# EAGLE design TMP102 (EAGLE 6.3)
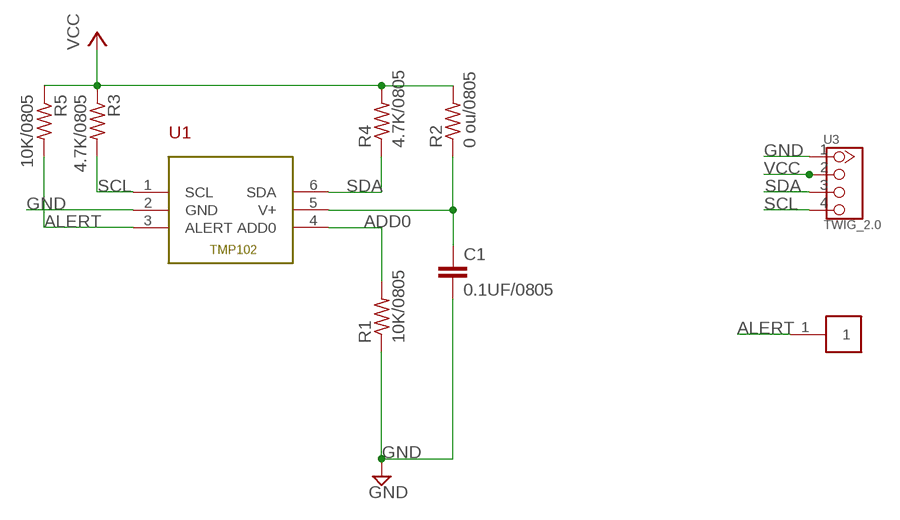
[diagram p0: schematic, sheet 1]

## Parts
C1  0.1UF/0805  C-EUC0805  [C0805]
R1  10K/0805  R-US_R0805  [R0805]
R2  0 ou/0805  R-US_R0805  [R0805]
R3  4.7K/0805  R-US_R0805  [R0805]
R4  4.7K/0805  R-US_R0805  [R0805]
R5  10K/0805  R-US_R0805  [R0805]
U1  TMP102  [TMP102]
U3  TWIG_2.0  [2.0_1X4]
U$1  PIN-1-2.0  [PIN-1-2.0]

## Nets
ADD0: R1.2 U1.4(ADD0)
ALERT: R5.2 U1.3(ALERT) U$1.1
GND: C1.2 R1.1 U1.2(GND) U3.1
N$6: C1.1 R2.1 U1.5(V+)
SCL: R3.2 U1.1(SCL) U3.4
SDA: R4.1 U1.6(SDA) U3.3
VCC: R2.2 R3.1 R4.2 R5.1 U3.2

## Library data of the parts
C1 = resistor:C-EU: CAPACITOR, European symbol
R1-R5 = resistor:R-US_: RESISTOR, American symbol
U1 = TMP102:TMP102
U3 = CONNECTER:TWIG_2.0
U$1 = PIN-1-2.0:PIN-1-2.0

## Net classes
0 default: width 0.003 mm, drill 0.254 mm, clearance 0.152 mm

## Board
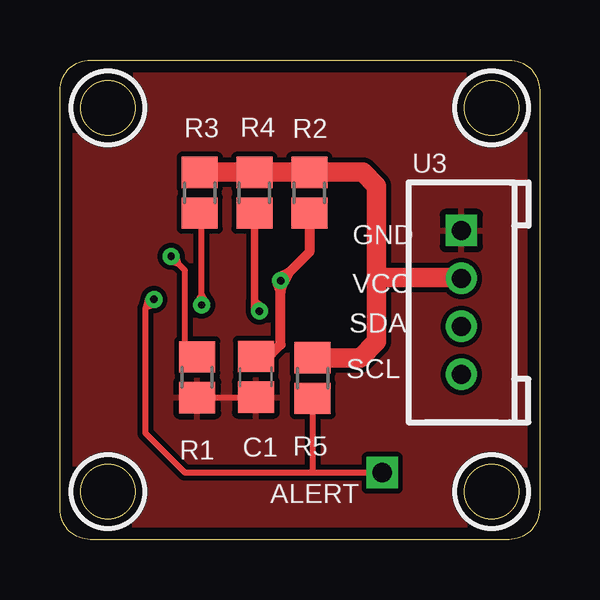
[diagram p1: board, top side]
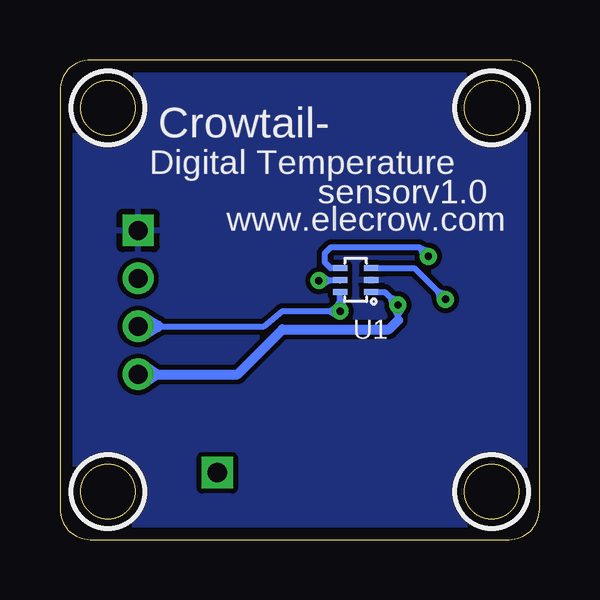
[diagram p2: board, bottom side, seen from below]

Size 20 x 20 mm. Coordinates in mm from the lower left corner, seen from the top.
Outline: 0,1.27 0,18.73 arc-90 1.27,20 18.73,20 arc-90 20,18.73 20,1.27 arc-90 18.73,0 1.27,0 arc-90 0,1.27
Outline: circle at 18,18 radius 1.14
Outline: circle at 18,2 radius 1.14
Outline: circle at 2,18 radius 1.14
Outline: circle at 2,2 radius 1.14
Copper layers (1*16): Top 0.035mm / dielectric 1.5mm / Bottom 0.035mm
Design rules "default *": minimum track width 10mil, minimum drill 12mil, track to track 8mil, track to pad 8mil, pad to pad 8mil, via to via 8mil, smd to smd 8mil, copper to edge 20mil, drill to drill 8mil, minimum pad ring 10mil, minimum via ring 8mil, stop-mask expansion 2mil, vias tented up to drill 100mil, thermal gap 10mil
tRestrict: area 16.5,16.5 to 19.5,19.5; area 16.5,0.5 to 19.5,3.5; area 0.5,16.5 to 3.5,19.5; area 0.5,0.5 to 3.5,3.5
bRestrict: area 16.5,16.5 to 19.5,19.5; area 16.5,0.5 to 19.5,3.5; area 0.5,16.5 to 3.5,19.5; area 0.5,0.5 to 3.5,3.5

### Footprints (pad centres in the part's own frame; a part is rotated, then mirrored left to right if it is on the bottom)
C0805 = smd 1.3 x 1.5: 1 -0.85,0; 2 0.85,0
R0805 = smd 1.3 x 1.5: 1 -0.85,0; 2 0.85,0
TMP102 = smd 0.6 x 0.25: 1 0,0; 2 0,-0.5; 3 0,-1; 4 1.3,-1; 5 1.3,-0.5; 6 1.3,0
2.0_1X4 = drill 0.8 pad 1.27 square: 1 -3,0 | drill 0.8 pad 1.27: 2 -1,0; 3 1,0; 4 3,0
PIN-1-2.0 = drill 0.8 square: 1 0,0

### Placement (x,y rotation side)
C1  8.17,6.79 270 top
R1  5.72,6.77 90 top
R2  10.4,14.46 90 top
R3  5.83,14.46 270 top
R4  8.11,14.46 90 top
R5  10.54,6.73 270 top
U1  7.02,10.32 180 bottom
U3  16.74,9.89 270 top
U$1  13.44,2.79 0 top

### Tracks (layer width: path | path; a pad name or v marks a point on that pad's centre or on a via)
ADD0  (via drill 0.3)
  Top 0.254: 6.28,7.49 6.1,7.49 R1.2 arc-90 5.21,8.13 5.21,11.24 4.96,11.49 | 4.96,11.49 4.85,11.87 v4.63,11.81 | 4.96,11.49 4.57,11.59
  Bottom 0.254: U1.4 8.71,11.32 8.95,11.56 8.95,11.94 8.7,12.19 5.01,12.19 4.96,12.13 | 4.96,12.13 4.57,12.03 | 4.96,12.13 4.85,11.75 v4.63,11.81
ALERT  (via drill 0.3)
  Top 0.254: U$1.1 10.54,2.79 | 10.54,2.79 5.21,2.79 3.56,4.45 3.56,9.65 3.6,9.69 | v3.92,10.02 3.6,9.69 | R5.2 10.54,2.79 | 3.6,9.69 3.98,9.79 v3.92,10.02 | 3.6,9.69 3.7,10.07 v3.92,10.02
  Bottom 0.254: 4.24,10.34 5.22,11.32 U1.3 | 4.24,10.34 v3.92,10.02 3.86,10.24 4.24,10.34 | 4.24,10.34 4.14,9.96
GND
  Top 0.254: R1.1 8.15,5.92 arc90 C1.2
  pour Bottom: -0.89,-0.51 -0.89,20.57 20.57,20.57 20.57,-0.51
  pour Top: -0.89,-0.51 -0.89,20.57 20.57,20.57 20.57,-0.51
N$6  (via drill 0.3)
  Top 0.406: C1.1 8.81,7.73 9.21,8.13 9.21,10.34 | 9.21,10.34 v9.21,10.79 | R2.1 10.4,11.99 9.53,11.12 | 9.53,11.12 v9.21,10.79 | 9.21,10.34 9.35,10.74 v9.21,10.79 | 9.21,10.34 9.06,10.74 v9.21,10.79 | 9.53,11.12 9.14,10.93 v9.21,10.79 | 9.53,11.12 9.34,10.73 v9.21,10.79
  Bottom 0.254: U1.5 8.32,10.79 8.75,10.79 | 8.75,10.79 v9.21,10.79 | 8.75,10.79 9.09,10.6 v9.21,10.79 | 8.75,10.79 9.09,10.99 v9.21,10.79
SCL  (via drill 0.3)
  Top 0.254: v5.9,9.78 5.9,10.24 | 5.9,10.24 5.9,13.54 R3.2 | 5.9,10.24 5.71,9.89 v5.9,9.78 | 5.9,10.24 6.1,9.89 v5.9,9.78
  Bottom 0.254: v5.9,9.78 5.9,9.32 | 5.9,9.32 5.9,9.14 | U1.1 6.44,10.32 6.23,10.1 | 6.23,10.1 v5.9,9.78 | 5.9,9.32 6.1,9.66 v5.9,9.78 | 5.9,9.32 5.71,9.66 v5.9,9.78 | 6.23,10.1 5.84,10 v5.9,9.78 | 6.23,10.1 6.12,9.72 v5.9,9.78
  Bottom 0.406: U3.4 15.94,6.89 | 15.94,6.89 12.6,6.89 10.73,8.76 6.28,8.76 5.9,9.14 | 15.94,6.89 16.49,6.52 U3.4 | 15.94,6.89 16.49,7.26 U3.4
SDA  (via drill 0.3)
  Top 0.305: R4.1 8.11,9.93 | 8.11,9.93 8.11,9.73 v8.32,9.53 | 8.11,9.93 8.11,9.53 v8.32,9.53 | 8.11,9.93 8.44,9.69 v8.32,9.53
  Bottom 0.254: v8.32,9.53 8.32,9.98 | 8.32,9.98 U1.6 | U3.3 15.94,8.89 11.49,8.89 10.73,9.53 8.77,9.53 | 8.77,9.53 v8.32,9.53 | 8.32,9.98 8.12,9.64 v8.32,9.53 | 8.32,9.98 8.51,9.64 v8.32,9.53 | 8.77,9.53 8.43,9.72 v8.32,9.53 | 8.77,9.53 8.43,9.33 v8.32,9.53
  Bottom 0.508: 15.94,8.89 16.54,8.54 U3.3 16.54,9.23 15.94,8.89
VCC
  Top 0.813: R3.1 R4.2 R2.2 12.63,15.31 13.21,14.73 13.21,10.92 | 13.21,10.92 16.71,10.92 U3.2 | R5.1 12.53,7.58 13.21,8.25 13.21,10.92

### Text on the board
bPlace: Crowtail- | Digital Temperature | sensorv1.0 | www.elecrow.com | U1
tNames: GND | VCC | SDA | SCL | ALERT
